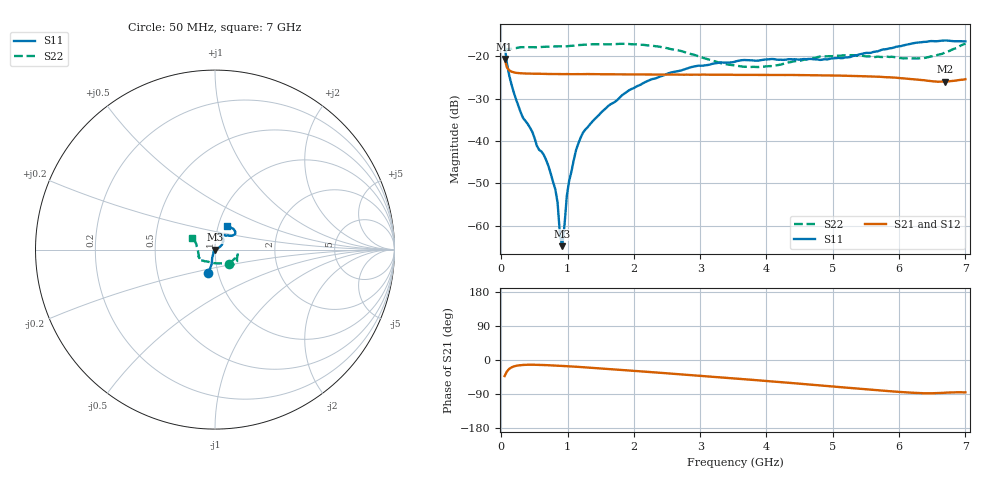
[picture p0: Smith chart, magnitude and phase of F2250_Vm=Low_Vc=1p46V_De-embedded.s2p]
! Integrated Device Technology
! Corporate Headquarters
! 6024 Silver Creek Valley Road
! San Jose, CA 95138  USA
! Phone:  1-408-284-8200
! Toll Free:  1-800-223-1366
! Webpage:  http://www.idt.com/
! Timing and RF Division
! 515 Groton Road, Suite 102
! Westford, MA 01886-6024
! Device:  F2250
! Description: Voltage Variable RF Attenuator
! Frequency:  50.0 -  6000.00 MHz
! Package:  3x3 mm Thin QFN Plastic Package: 16 pin
! Ports:  2 RF, 3 DC
!  Pin  1  = GND
!  Pin  2  = NC
!  Pin  3  = RF1  = Port 1
!  Pin  4  = NC
!  Pin  5  = GND
!  Pin  6  = GND
!  Pin  7  = GND
!  Pin  8  = GND
!  Pin  9  = NC
!  Pin 10  = RF2  = Port 2
!  Pin 11  = NC
!  Pin 12  = GND
!  Pin 13  = GND
!  Pin 14  = VCNTRL
!  Pin 15  = VDD
!  Pin 16  = VMODE
! Vcntrl:  1.460 Volts
! Vmode:  +0.000 Volts
! Vdd:  +3.30  Volts
! Current:  1.191 mA
! Data:  The device was measured on a the F2250 evaluation board which has
!  individual transmission lines to the RF pins.  Data was collected
!  using a calibrated network analyzer.  The evaluation board was
!  de-embedded using a TRL calibration technique.
!  The reference plane is the edge of the package pin.
! Misc:  SN 10
!  Action Tracker AT0258
! Date Measured:  2014-11-26
! Date:  2015-10-15  MJV
! Note:
!  Integrated Device Technology supplies this data as a sample of measured
!  data at the package pin for this product.  Your particular data for this
!  product may vary.
!  Data was taken at 25 degrees C.
!  Integrated Device Technology reserves the right to change this data at anytime.
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# GHz S dB R 50
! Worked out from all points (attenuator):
!   201 points, 50 MHz to 7 GHz, reference 50 ohm
!   highest |S21| = -20.61 dB at 50 MHz (marker M1); lowest = -26.0 dB at 6.687 GHz (marker M2)
!   lowest |S11| = -64.8 dB at 918.8 MHz (marker M3), VSWR 1.00, Z = 50 + j0.0556 ohm
!   |S11| at or under -10 dB: start of sweep to end of sweep
!   |S22| runs from -22.5 to -16.9 dB; largest |S21 - S12| = 0.00022
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0.05  -17.29 -105.6  -20.61 -42.5  -20.60 -42.4  -18.98 -45.2
0.1195  -24.48 -105.8  -23.28 -23.4  -23.29 -23.4  -18.26 -16.7
0.22375  -30.19 -111.5  -23.87 -15.4  -23.86 -15.4  -18.03 -12.5
0.5365  -41.10 -130.9  -24.10 -12.7  -24.08 -12.7  -17.84 -14.0
0.6755  -44.43 -132.4  -24.15 -13.5  -24.15 -13.5  -17.71 -16.4
0.8145  -51.36 -167.3  -24.17 -14.7  -24.18 -14.7  -17.65 -19.3
0.84925  -54.56 -166.4  -24.16 -15.0  -24.17 -15.0  -17.63 -20.1
0.884  -61.94 -173.9  -24.16 -15.3  -24.17 -15.3  -17.61 -20.9
0.91875  -64.81 104.6  -24.17 -15.6  -24.16 -15.6  -17.60 -21.7
0.9535  -59.83 -75.6  -24.18 -16.0  -24.16 -16.0  -17.68 -22.1
0.98825  -52.94 -18.0  -24.16 -16.3  -24.17 -16.3  -17.59 -22.5
1.023  -49.39 -5.3  -24.18 -16.7  -24.18 -16.7  -17.54 -22.7
1.12725  -42.14 12.1  -24.18 -17.8  -24.18 -17.8  -17.38 -24.5
1.2315  -38.03 16.8  -24.18 -19.0  -24.17 -19.0  -17.23 -26.5
1.82225  -29.16 29.8  -24.22 -26.4  -24.23 -26.4  -17.02 -32.9
2.37825  -24.85 41.3  -24.28 -33.5  -24.28 -33.5  -17.68 -38.7
3.525  -21.23 69.7  -24.36 -48.9  -24.36 -48.9  -22.13 -81.0
4.081  -20.60 77.3  -24.38 -56.5  -24.39 -56.5  -22.29 -116.8
4.7065  -20.68 70.9  -24.42 -65.6  -24.42 -65.6  -20.38 -140.1
5.85325  -18.12 38.9  -24.94 -82.3  -24.93 -82.3  -20.13 -157.5
6.68725  -16.23 47.9  -25.98 -86.4  -25.99 -86.4  -19.10 162.2
7  -16.44 62.7  -25.38 -85.4  -25.40 -85.4  -16.95 153.7
